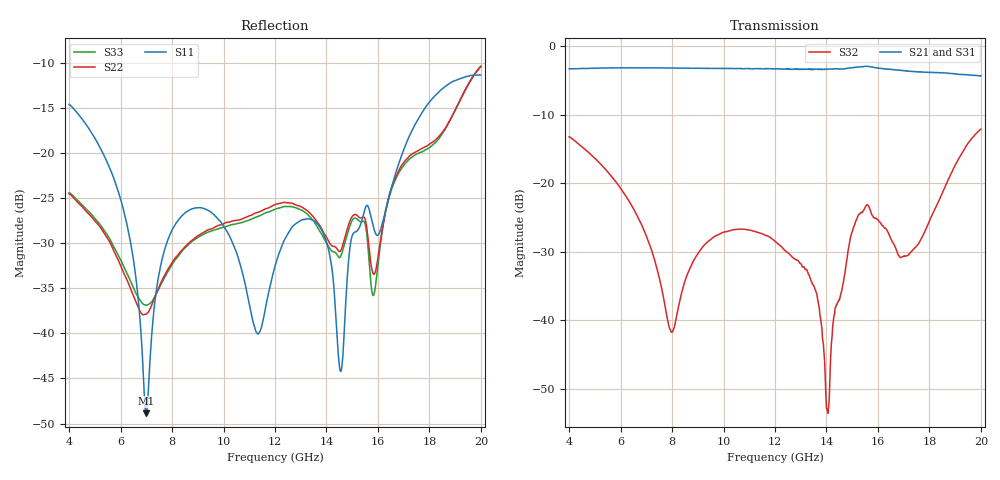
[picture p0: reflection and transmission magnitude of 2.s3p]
!The following data was pulled from an Agilent PNA
!This sNp file was generated from the data in the RF Test software
!NOTE:  Smoothing/Math/Corrections applied on any given trace ARE included in the data saved here
# MHz S dB R 50
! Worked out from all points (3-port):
!   1601 points, 4 GHz to 20 GHz, reference 50 ohm
!   strongest paths, dB at 4 GHz, 8 GHz, 12 GHz, 16 GHz, 20 GHz:
!     S21: -3.3, -3.2, -3.3, -3.2, -4.3
!     S31: -3.3, -3.2, -3.3, -3.2, -4.3
!     S32: -13.2, -41.7, -28.4, -25.3, -12.1
!   lowest |S11| = -48.9 dB at 7 GHz (marker M1), VSWR 1.01, Z = 50.1 - j0.355 ohm
!   |S11| at or under -10 dB: start of sweep to end of sweep
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4000  -14.63 90.4  -3.29 -108.6  -3.29 -108.9
      -3.29 -108.5  -24.53 -57.3  -13.21 -139.2
      -3.29 -108.8  -13.21 -139.2  -24.42 -57.9
6100  -26.17 35.2  -3.15 -169.3  -3.16 -169.8
      -3.14 -169.3  -33.15 -123.8  -21.25 165.5
      -3.14 -169.8  -21.25 165.5  -32.45 -124.7
7000  -48.87 -80.3  -3.15 163.9  -3.16 163.3
      -3.15 163.9  -37.85 -90.6  -27.69 146.2
      -3.17 163.4  -27.68 146.3  -36.86 -99.6
8350  -27.07 160.1  -3.18 122.9  -3.18 122.2
      -3.19 122.8  -30.89 -68.2  -36.31 -119.3
      -3.19 122.1  -36.31 -119.3  -31.02 -73.5
12000  -32.56 -106.1  -3.28 4.9  -3.31 4.0
       -3.30 5.1  -25.74 -88.4  -28.43 167.9
       -3.30 4.2  -28.43 167.9  -26.24 -91.4
14040  -30.26 140.8  -3.33 -66.9  -3.36 -67.6
       -3.36 -66.8  -29.56 -104.6  -53.56 -170.5
       -3.37 -67.7  -53.22 -171.9  -30.18 -107.5
14550  -44.21 54.6  -3.29 -85.8  -3.31 -86.6
       -3.29 -86.0  -30.87 -81.5  -36.22 -105.1
       -3.37 -86.3  -36.24 -104.9  -31.47 -84.2
15190  -28.64 -132.6  -3.04 -110.7  -3.02 -111.9
       -3.04 -110.7  -26.92 -85.7  -25.08 -126.8
       -3.02 -111.8  -25.09 -126.7  -27.34 -88.9
16830  -21.02 -41.9  -3.47 179.3  -3.50 178.2
       -3.50 179.5  -21.82 -67.9  -30.60 172.5
       -3.56 178.4  -30.64 172.7  -22.11 -69.3
20000  -11.38 162.8  -4.50 39.4  -4.49 38.2
       -4.29 38.9  -10.44 34.3  -12.05 158.1
       -4.32 37.8  -12.09 158.3  -10.39 33.5
